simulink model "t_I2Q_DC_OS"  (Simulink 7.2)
settings: Solver=ode3  SolverMode=SingleTasking  StartTime=0.0  StopTime=0.01  FixedStep=10e-6  MaxStep=5e-6  RelTol=1e-6  AbsTol=1e-6

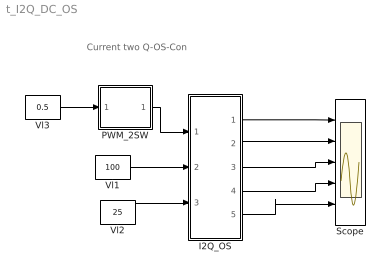
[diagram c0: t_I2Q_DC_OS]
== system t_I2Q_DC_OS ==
  note: Current two Q-OS-Con
  I2Q_OS : Subsystem  mask{L=5e-3, IL0=30, C=2e-4, VC0=50, R=10}
      mask prompts: L "Inductance L"; IL0 "Initial Ind. Current"; C "Capacitance"; VC0 "Initial Cap. Voltage"; R "Load Resistance"
      mask help: Current two Quadrant Converter Input Vector u: u[0]= T1.gate u[1]= T2.gate u[2]= E.v u[3]= IDC.i Output Vector y: y[0]= T1.I y[1]= T1.V y[2]= T2.I y[3]= T2.V y[4]= L1.I y[5]= C1.V y[6]= E.I Parameter Vector p: p[0]= L1.L p[1]= L1.iL0 p[2]= C1.C p[3]= C1.vC0 p[4]= R1.r You can pause the simulation during running, change the Parameters you want and continue the Simulation
  PWM_2SW : Subsystem  mask(PWM-2L-1PH){FT=2000, PHT=0, DT=1e-6}
      mask prompts: FT "Triangular Frequency"; PHT "Trian. Phase Angle (Degree)"; DT "Dead Time"
      mask help: Pulse Width Modulation for 1 Phase Converter
  Scope : Scope  NumInputPorts=5
  Vl1 : Constant  Value=100
  Vl2 : Constant  Value=25
  Vl3 : Constant  Value=0.5
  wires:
  I2Q_OS/1("iT1, iD1") -> Scope/1
  I2Q_OS/2("iT2, iD2") -> Scope/2
  Vl1/1 -> I2Q_OS/2(E)
  Vl2/1 -> I2Q_OS/3(iDC)
  I2Q_OS/3(iL1) -> Scope/3
  I2Q_OS/4(vC) -> Scope/4
  Vl3/1 -> PWM_2SW/1(In1)
  PWM_2SW/1(Out1) -> I2Q_OS/1(sw)
  I2Q_OS/5(iE) -> Scope/5

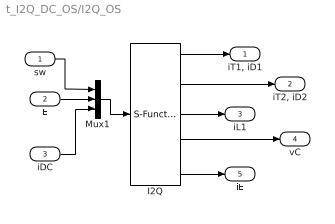
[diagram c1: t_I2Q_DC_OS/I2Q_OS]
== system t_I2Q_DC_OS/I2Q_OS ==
  sw : Inport  OutDataType=sfix(16)  OutScaling=2^0
  E : Inport  Port=2  OutDataType=sfix(16)  OutScaling=2^0
  iDC : Inport  Port=3  OutDataType=sfix(16)  OutScaling=2^0
  I2Q : S-Function  FunctionName=s_I2Q_DC_OS  Parameters="[L  IL0 C  VC0  R]"  EnableBusSupport=off
  Mux1 : Mux  Inputs=3
  "iT1, iD1" : Outport  OutDataType=sfix(16)  OutScaling=2^0
  "iT2, iD2" : Outport  Port=2  OutDataType=sfix(16)  OutScaling=2^0
  iL1 : Outport  Port=3  OutDataType=sfix(16)  OutScaling=2^0
  vC : Outport  Port=4  OutDataType=sfix(16)  OutScaling=2^0
  iE : Outport  Port=5  OutDataType=sfix(16)  OutScaling=2^0
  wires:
  Mux1/1 -> I2Q/1
  sw/1 -> Mux1/1
  E/1 -> Mux1/2
  I2Q/1 -> "iT1, iD1"/1
  I2Q/2 -> "iT2, iD2"/1
  iDC/1 -> Mux1/3
  I2Q/4 -> vC/1
  I2Q/3 -> iL1/1
  I2Q/5 -> iE/1

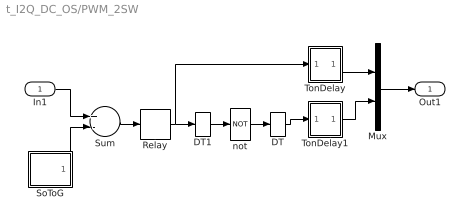
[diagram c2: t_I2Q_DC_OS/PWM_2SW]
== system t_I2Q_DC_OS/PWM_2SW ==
  In1 : Inport  OutDataType=sfix(16)  OutScaling=2^0
  DT : DataTypeConversion
  DT1 : DataTypeConversion
  Mux : Mux  Inputs=2
  Relay : Relay  OutDataType=sfix(16)  OutScaling=2^0
  SoToG : Subsystem  mask(SoToG){T=1e-3}
      mask prompts: T "Period Time"
  Sum : Sum  Inputs=+-  OutDataType=sfix(16)  OutScaling=2^0
  TonDelay : Subsystem  mask(TonDelay){DT=DT}
      mask prompts: DT "Dead Time"
      mask help: Turn on dead time to protect against short circuit of the converter leg
  TonDelay1 : Subsystem  mask(TonDelay){DT=DT}
      mask prompts: DT "Dead Time"
      mask help: Turn on dead time to protect against short circuit of the converter leg
  not : Logic  Operator=NOT  Inputs=1
  Out1 : Outport  InitialOutput=0
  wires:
  DT1/1 -> not/1
  DT/1 -> TonDelay1/1(s1)
  In1/1 -> Sum/1
  SoToG/1(O) -> Sum/2
  Sum/1 -> Relay/1
  not/1 -> DT/1
  TonDelay1/1(s1d) -> Mux/2
  Relay/1 -> DT1/1, TonDelay/1(s1)
  TonDelay/1(s1d) -> Mux/1
  Mux/1 -> Out1/1

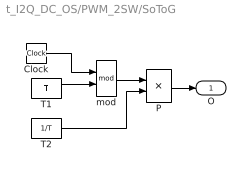
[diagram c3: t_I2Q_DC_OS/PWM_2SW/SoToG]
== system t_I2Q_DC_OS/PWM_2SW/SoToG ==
  Clock : Clock
  P : Product  OutDataType=sfix(16)  OutScaling=2^0
  T1 : Constant  Value=T  OutDataType=sfix(16)  OutScaling=2^0
  T2 : Constant  Value=1/T  OutDataType=sfix(16)  OutScaling=2^0
  mod : Math  Operator=mod
  O : Outport
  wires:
  Clock/1 -> mod/1
  T1/1 -> mod/2
  T2/1 -> P/2
  mod/1 -> P/1
  P/1 -> O/1

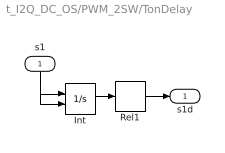
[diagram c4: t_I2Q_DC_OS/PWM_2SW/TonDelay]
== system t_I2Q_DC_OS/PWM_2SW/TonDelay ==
  s1 : Inport  Orientation=down  OutDataType=sfix(16)  OutScaling=2^0
  Int : Integrator  ExternalReset=falling
  Rel1 : Relay  OnSwitchValue=DT  OutDataType=sfix(16)  OutScaling=2^0
  s1d : Outport  InitialOutput=0
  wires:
  Int/1 -> Rel1/1
  s1/1 -> Int/2, Int/1
  Rel1/1 -> s1d/1

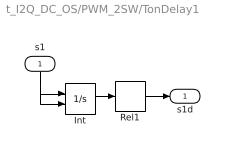
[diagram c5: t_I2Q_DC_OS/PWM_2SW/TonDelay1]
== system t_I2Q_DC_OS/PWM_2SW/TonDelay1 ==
  s1 : Inport  Orientation=down  OutDataType=sfix(16)  OutScaling=2^0
  Int : Integrator  ExternalReset=falling
  Rel1 : Relay  OnSwitchValue=DT  OutDataType=sfix(16)  OutScaling=2^0
  s1d : Outport  InitialOutput=0
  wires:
  Int/1 -> Rel1/1
  s1/1 -> Int/2, Int/1
  Rel1/1 -> s1d/1
